FUNCTION "CENTR. 4  POSTERIORE SX" : VOID
TITLE =
VERSION : 0.1

BEGIN
NETWORK
TITLE =LETTURA STATUS WORD DA DRIVE
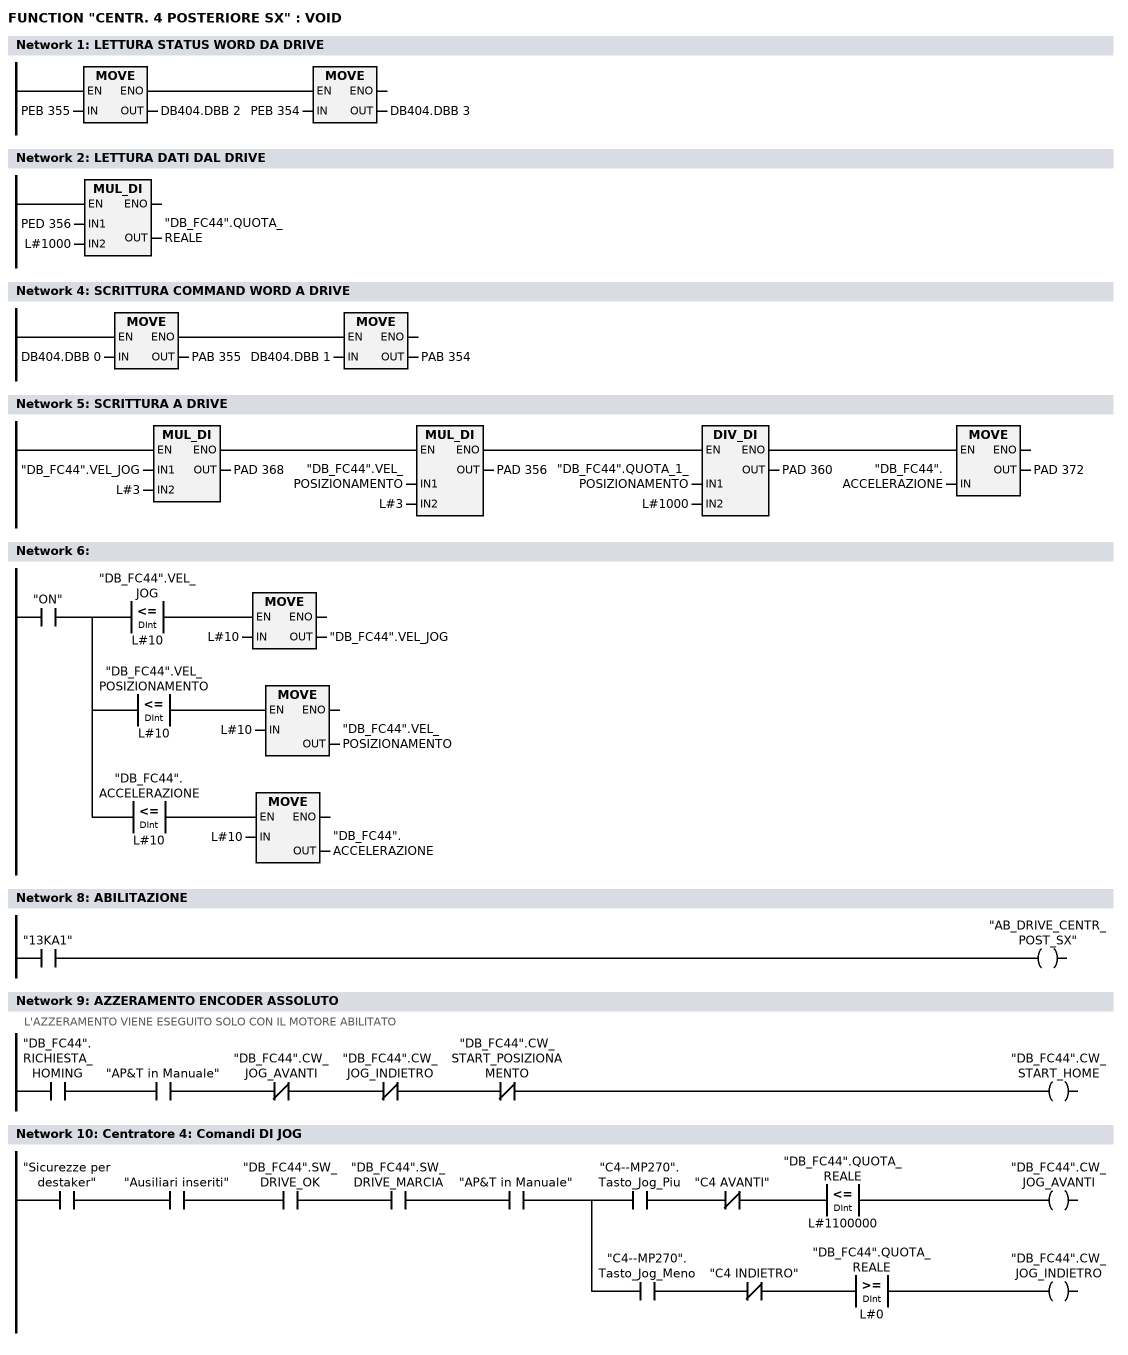
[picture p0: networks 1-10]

      U(    ;
      L     PEB  355;
      T     DB404.DBB    2;
      SET   ;
      SAVE  ;
      CLR   ;
      U     BIE;
      )     ;
      SPBNB _001;
      L     PEB  354;
      T     DB404.DBB    3;
_001: NOP   0;
NETWORK
TITLE =LETTURA DATI DAL DRIVE

      L     PED  356;
      L     L#1000;
      *D    ;
      T     "DB_FC44".QUOTA_REALE;
      NOP   0;
NETWORK
TITLE =

NETWORK
TITLE =SCRITTURA COMMAND WORD A DRIVE

      U(    ;
      L     DB404.DBB    0;
      T     PAB  355;
      SET   ;
      SAVE  ;
      CLR   ;
      U     BIE;
      )     ;
      SPBNB _002;
      L     DB404.DBB    1;
      T     PAB  354;
_002: NOP   0;
NETWORK
TITLE =SCRITTURA A DRIVE

      U(    ;
      U(    ;
      U(    ;
      L     "DB_FC44".VEL_JOG;
      L     L#3;
      *D    ;
      T     PAD  368;
      UN    OV;
      SAVE  ;
      CLR   ;
      U     BIE;
      )     ;
      SPBNB _003;
      L     "DB_FC44".VEL_POSIZIONAMENTO;
      L     L#3;
      *D    ;
      T     PAD  356;
      UN    OV;
      SAVE  ;
      CLR   ;
_003: U     BIE;
      )     ;
      SPBNB _004;
      L     "DB_FC44".QUOTA_1_POSIZIONAMENTO;
      L     L#1000;
      /D    ;
      T     PAD  360;
      UN    OV;
      SAVE  ;
      CLR   ;
_004: U     BIE;
      )     ;
      SPBNB _005;
      L     "DB_FC44".ACCELERAZIONE;
      T     PAD  372;
_005: NOP   0;
NETWORK
TITLE =

      U     "ON";
      =     L      0.0;
      U     L      0.0;
      U(    ;
      L     "DB_FC44".VEL_JOG;
      L     L#10;
      <=D   ;
      )     ;
      SPBNB _006;
      L     L#10;
      T     "DB_FC44".VEL_JOG;
_006: NOP   0;
      U     L      0.0;
      U(    ;
      L     "DB_FC44".VEL_POSIZIONAMENTO;
      L     L#10;
      <=D   ;
      )     ;
      SPBNB _007;
      L     L#10;
      T     "DB_FC44".VEL_POSIZIONAMENTO;
_007: NOP   0;
      U     L      0.0;
      U(    ;
      L     "DB_FC44".ACCELERAZIONE;
      L     L#10;
      <=D   ;
      )     ;
      SPBNB _008;
      L     L#10;
      T     "DB_FC44".ACCELERAZIONE;
_008: NOP   0;
NETWORK
TITLE =

NETWORK
TITLE =ABILITAZIONE

      U     "13KA1";
      =     "AB_DRIVE_CENTR_POST_SX";
NETWORK
TITLE =AZZERAMENTO ENCODER ASSOLUTO
//L'AZZERAMENTO VIENE ESEGUITO SOLO CON IL MOTORE ABILITATO
      U     "DB_FC44".RICHIESTA_HOMING;
      U     "AP&T in Manuale";
      UN    "DB_FC44".CW_JOG_AVANTI;
      UN    "DB_FC44".CW_JOG_INDIETRO;
      UN    "DB_FC44".CW_START_POSIZIONAMENTO;
      =     "DB_FC44".CW_START_HOME;
NETWORK
TITLE =Centratore 4: Comandi DI JOG

      U     "Sicurezze per destaker";
      U     "Ausiliari inseriti";
      U     "DB_FC44".SW_DRIVE_OK;
      U     "DB_FC44".SW_DRIVE_MARCIA;
      U     "AP&T in Manuale";
      =     L      0.0;
      U     L      0.0;
      U     "C4--MP270".Tasto_Jog_Piu;
      UN    "C4 AVANTI";
      U(    ;
      L     "DB_FC44".QUOTA_REALE;
      L     L#1100000;
      <=D   ;
      )     ;
      =     "DB_FC44".CW_JOG_AVANTI;
      U     L      0.0;
      U     "C4--MP270".Tasto_Jog_Meno;
      UN    "C4 INDIETRO";
      U(    ;
      L     "DB_FC44".QUOTA_REALE;
      L     L#0;
      >=D   ;
      )     ;
      =     "DB_FC44".CW_JOG_INDIETRO;
NETWORK
TITLE =Centratore 4: Posizioni

      U     "ON";
      =     L      0.0;
      U     L      0.0;
      U(    ;
      L     "DB_FC44".QUOTA_REALE;
      L     L#100;
      <=D   ;
      )     ;
      U(    ;
      L     "DB_FC44".QUOTA_REALE;
      L     L#-100;
      >=D   ;
      )     ;
      =     "C4: Asse in pos.0";
      U(    ;
      U(    ;
      U     L      0.0;
      SPBNB _009;
      L     "MATRICOLA ATTUALE".C4_Posizione_1;
      L     L#100;
      -D    ;
      T     "CONFRONTI CENTRATORI".C4_Pos_1_Min;
      UN    OV;
      SAVE  ;
      CLR   ;
_009: U     BIE;
      )     ;
      SPBNB _00a;
      L     "MATRICOLA ATTUALE".C4_Posizione_1;
      L     L#200;
      +D    ;
      T     "CONFRONTI CENTRATORI".C4_Pos_1_Max;
      UN    OV;
      SAVE  ;
      CLR   ;
_00a: U     BIE;
      )     ;
      U(    ;
      L     "DB_FC44".QUOTA_REALE;
      L     "CONFRONTI CENTRATORI".C4_Pos_1_Min;
      >=D   ;
      )     ;
      U(    ;
      L     "DB_FC44".QUOTA_REALE;
      L     "CONFRONTI CENTRATORI".C4_Pos_1_Max;
      <=D   ;
      )     ;
      =     "C4: Asse in pos.1";
      U(    ;
      U(    ;
      U     L      0.0;
      SPBNB _00b;
      L     "MATRICOLA ATTUALE".C4_Posizione_2;
      L     L#100;
      -D    ;
      T     "CONFRONTI CENTRATORI".C4_Pos_2_Min;
      UN    OV;
      SAVE  ;
      CLR   ;
_00b: U     BIE;
      )     ;
      SPBNB _00c;
      L     "MATRICOLA ATTUALE".C4_Posizione_2;
      L     L#50000;
      +D    ;
      T     "CONFRONTI CENTRATORI".C4_Pos_2_Max;
      UN    OV;
      SAVE  ;
      CLR   ;
_00c: U     BIE;
      )     ;
      U(    ;
      L     "DB_FC44".QUOTA_REALE;
      L     "CONFRONTI CENTRATORI".C4_Pos_2_Min;
      >=D   ;
      )     ;
      UN    "C4: Asse in pos.3";
      UN    "C4: Asse in pos.4";
      =     "C4: Asse in pos.2";
      U(    ;
      U(    ;
      U     L      0.0;
      SPBNB _00d;
      L     "MATRICOLA ATTUALE".C4_Posizione_3;
      L     L#100;
      -D    ;
      T     "CONFRONTI CENTRATORI".C4_Pos_3_Min;
      UN    OV;
      SAVE  ;
      CLR   ;
_00d: U     BIE;
      )     ;
      SPBNB _00e;
      L     "MATRICOLA ATTUALE".C4_Posizione_3;
      L     L#50000;
      +D    ;
      T     "CONFRONTI CENTRATORI".C4_Pos_3_Max;
      UN    OV;
      SAVE  ;
      CLR   ;
_00e: U     BIE;
      )     ;
      U(    ;
      L     "DB_FC44".QUOTA_REALE;
      L     "CONFRONTI CENTRATORI".C4_Pos_3_Min;
      >=D   ;
      )     ;
      UN    "C4: Asse in pos.4";
      =     "C4: Asse in pos.3";
      U(    ;
      U(    ;
      U     L      0.0;
      SPBNB _00f;
      L     "MATRICOLA ATTUALE".C4_Posizione_4;
      L     L#100;
      -D    ;
      T     "CONFRONTI CENTRATORI".C4_Pos_4_Min;
      UN    OV;
      SAVE  ;
      CLR   ;
_00f: U     BIE;
      )     ;
      SPBNB _010;
      L     "MATRICOLA ATTUALE".C4_Posizione_4;
      L     L#100;
      +D    ;
      T     "CONFRONTI CENTRATORI".C4_Pos_4_Max;
      UN    OV;
      SAVE  ;
      CLR   ;
_010: U     BIE;
      )     ;
      U(    ;
      L     "DB_FC44".QUOTA_REALE;
      L     "CONFRONTI CENTRATORI".C4_Pos_4_Min;
      >=D   ;
      )     ;
      U(    ;
      L     "DB_FC44".QUOTA_REALE;
      L     "CONFRONTI CENTRATORI".C4_Pos_4_Max;
      <=D   ;
      )     ;
      =     "C4: Asse in pos.4";
NETWORK
TITLE =Centratore 4: consenso abilitazione passi
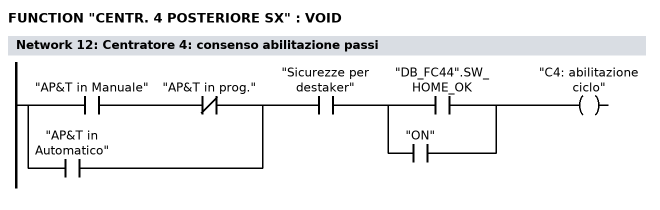
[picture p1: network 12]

      U(    ;
      U     "AP&T in Manuale";
      UN    "AP&T in prog.";
      O     "AP&T in Automatico";
      )     ;
      U     "Sicurezze per destaker";
      U(    ;
      O     "DB_FC44".SW_HOME_OK;
      O     "ON";
      )     ;
      =     "C4: abilitazione ciclo";
NETWORK
TITLE =Centratore 4: comando avvicinamento  (centraggi aperti)

      U(    ;
      U(    ;
      O     "Comando apre centraggi";
      O     "C4--MP270".Tasto_Indietro;
      O     ;
      U     "Apertura centratori";
      U(    ;
      O     "Centratori a riposo";
      O     "Centratori tutti chiusi";
      )     ;
      )     ;
      UN    "C4: Asse in pos.1";
      UN    "C4: comando arrivo";
      UN    "C4: comando a riposo";
      U     "C4: abilitazione ciclo";
      L     S5T#100MS;
      SE    T    190;
      NOP   0;
      NOP   0;
      NOP   0;
      U     T    190;
      )     ;
      S     "C4: comando avvicinam";
      U(    ;
      O     "C4: Asse in pos.1";
      O(    ;
      U(    ;
      O     "Ripristino centratori";
      O     "Comando riposo centraggi";
      O     "C4--MP270".Tasto_Riposo;
      )     ;
      FP    "C4: one shot 1";
      )     ;
      )     ;
      R     "C4: comando avvicinam";
      NOP   0;
NETWORK
TITLE =Centratore 4: comando arrivo (centraggi chiusi)

      U(    ;
      U(    ;
      O     "Comando chiude centraggi";
      O     "C4--MP270".Tasto_Avanti;
      O     ;
      U     "Chiusura centratori";
      U(    ;
      O     "Centratori tutti aperti";
      O     "Centratori a riposo";
      )     ;
      )     ;
      UN    "C4: Asse in pos.4";
      UN    "C4: comando avvicinam";
      UN    "C4: comando a riposo";
      U     "C4: abilitazione ciclo";
      L     S5T#100MS;
      SE    T    191;
      NOP   0;
      NOP   0;
      NOP   0;
      U     T    191;
      )     ;
      S     "C4: comando arrivo";
      U(    ;
      O     "C4: Asse in pos.4";
      O(    ;
      U(    ;
      O     "Ripristino centratori";
      O     "Comando riposo centraggi";
      O     "C4--MP270".Tasto_Riposo;
      )     ;
      FP    "C4: one shot 2";
      )     ;
      )     ;
      R     "C4: comando arrivo";
      NOP   0;
NETWORK
TITLE =Centratore 4: comando automatico centraggi a riposo

      U(    ;
      U(    ;
      O     "Comando riposo centraggi";
      O     "C4--MP270".Tasto_Riposo;
      )     ;
      UN    "C4: Asse in pos.0";
      UN    "C4: comando avvicinam";
      UN    "C4: comando arrivo";
      U     "C4: abilitazione ciclo";
      L     S5T#100MS;
      SE    T    192;
      NOP   0;
      NOP   0;
      NOP   0;
      U     T    192;
      )     ;
      S     "C4: comando a riposo";
      U(    ;
      O     "C4: Asse in pos.0";
      O(    ;
      U     "Ripristino centratori";
      FP    "C4: one shot 3";
      )     ;
      )     ;
      R     "C4: comando a riposo";
      NOP   0;
NETWORK
TITLE =Centratore 4: quote impostate per posizioni

      U     "ON";
      =     L      0.0;
      U(    ;
      U(    ;
      U     L      0.0;
      U     "C4: comando a riposo";
      UN    "C4: Asse in pos.0";
      SPBNB _011;
      L     0;
      T     "DB_FC44".QUOTA_1_POSIZIONAMENTO;
      SET   ;
      SAVE  ;
      CLR   ;
_011: U     BIE;
      )     ;
      SPBNB _012;
      L     L#150;
      T     "DB_FC44".VEL_POSIZIONAMENTO;
      SET   ;
      SAVE  ;
      CLR   ;
_012: U     BIE;
      )     ;
      SPBNB _013;
      L     L#1000;
      T     "DB_FC44".ACCELERAZIONE;
      SET   ;
      SAVE  ;
      CLR   ;
_013: U     BIE;
      =     "C4: Quote pronte pos.0";
      U(    ;
      U(    ;
      U     L      0.0;
      U     "C4: comando avvicinam";
      UN    "C4: Asse in pos.1";
      SPBNB _014;
      L     "MATRICOLA ATTUALE".C4_Posizione_1;
      T     "DB_FC44".QUOTA_1_POSIZIONAMENTO;
      SET   ;
      SAVE  ;
      CLR   ;
_014: U     BIE;
      )     ;
      SPBNB _015;
      L     "MATRICOLA ATTUALE".C4_Velocita_1;
      T     "DB_FC44".VEL_POSIZIONAMENTO;
      SET   ;
      SAVE  ;
      CLR   ;
_015: U     BIE;
      )     ;
      SPBNB _016;
      L     "MATRICOLA ATTUALE".C4_Accell_1;
      T     "DB_FC44".ACCELERAZIONE;
      SET   ;
      SAVE  ;
      CLR   ;
_016: U     BIE;
      =     "C4: Quote pronte pos.1";
      U     L      0.0;
      U     "C4: comando arrivo";
      =     L      0.1;
      U(    ;
      U(    ;
      U     L      0.1;
      UN    "C4: Asse in pos.2";
      SPBNB _017;
      L     "MATRICOLA ATTUALE".C4_Posizione_4;
      T     "DB_FC44".QUOTA_1_POSIZIONAMENTO;
      SET   ;
      SAVE  ;
      CLR   ;
_017: U     BIE;
      )     ;
      SPBNB _018;
      L     "MATRICOLA ATTUALE".C4_Velocita_2;
      T     "DB_FC44".VEL_POSIZIONAMENTO;
      SET   ;
      SAVE  ;
      CLR   ;
_018: U     BIE;
      )     ;
      SPBNB _019;
      L     "MATRICOLA ATTUALE".C4_Accell_2;
      T     "DB_FC44".ACCELERAZIONE;
      SET   ;
      SAVE  ;
      CLR   ;
_019: U     BIE;
      S     "C4: Quote pronte pos.2";
      U     L      0.1;
      U     "C4: Quote pronte pos.2";
      UN    "C4: Reset start pos.2";
      L     S5T#1S;
      SE    "C4: ritardo P2";
      NOP   0;
      NOP   0;
      NOP   0;
      U     "C4: ritardo P2";
      S     "C4: Reset start pos.2";
      R     "C4: Quote pronte pos.2";
      U     L      0.0;
      U     "C4: comando arrivo";
      =     L      0.1;
      U(    ;
      U(    ;
      U(    ;
      U     L      0.1;
      U     "C4: Asse in pos.2";
      UN    "C4: Asse in pos.3";
      SPBNB _01a;
      L     "MATRICOLA ATTUALE".C4_Posizione_4;
      T     "DB_FC44".QUOTA_1_POSIZIONAMENTO;
      SET   ;
      SAVE  ;
      CLR   ;
_01a: U     BIE;
      )     ;
      SPBNB _01b;
      L     "MATRICOLA ATTUALE".C4_Velocita_3;
      T     "DB_FC44".VEL_POSIZIONAMENTO;
      SET   ;
      SAVE  ;
      CLR   ;
_01b: U     BIE;
      )     ;
      SPBNB _01c;
      L     "MATRICOLA ATTUALE".C4_Accell_3;
      T     "DB_FC44".ACCELERAZIONE;
      SET   ;
      SAVE  ;
      CLR   ;
_01c: U     BIE;
      )     ;
      U     "C4: Reset start pos.2";
      S     "C4: Quote pronte pos.3";
      R     "C4: Reset start pos.2";
      U     L      0.1;
      U     "C4: Quote pronte pos.3";
      L     S5T#500MS;
      SE    "C4: ritardo P3";
      NOP   0;
      NOP   0;
      NOP   0;
      U     "C4: ritardo P3";
      S     "C4: Reset start pos.3";
      R     "C4: Quote pronte pos.3";
      U     L      0.0;
      U     "C4: comando arrivo";
      =     L      0.1;
      U(    ;
      U(    ;
      U(    ;
      U     L      0.1;
      U     "C4: Asse in pos.3";
      UN    "C4: Asse in pos.4";
      SPBNB _01d;
      L     "MATRICOLA ATTUALE".C4_Posizione_4;
      T     "DB_FC44".QUOTA_1_POSIZIONAMENTO;
      SET   ;
      SAVE  ;
      CLR   ;
_01d: U     BIE;
      )     ;
      SPBNB _01e;
      L     "MATRICOLA ATTUALE".C4_Velocita_4;
      T     "DB_FC44".VEL_POSIZIONAMENTO;
      SET   ;
      SAVE  ;
      CLR   ;
_01e: U     BIE;
      )     ;
      SPBNB _01f;
      L     "MATRICOLA ATTUALE".C4_Accell_4;
      T     "DB_FC44".ACCELERAZIONE;
      SET   ;
      SAVE  ;
      CLR   ;
_01f: U     BIE;
      )     ;
      U     "C4: Reset start pos.3";
      S     "C4: Quote pronte pos.4";
      R     "C4: Reset start pos.3";
      U     L      0.1;
      U     "C4: Quote pronte pos.4";
      L     S5T#500MS;
      SE    "C4: ritardo P4";
      NOP   0;
      NOP   0;
      NOP   0;
      U     "C4: ritardo P4";
      S     "C4: Reset start pos.4";
      R     "C4: Quote pronte pos.4";
NETWORK
TITLE =Centratore 4: reset impostate
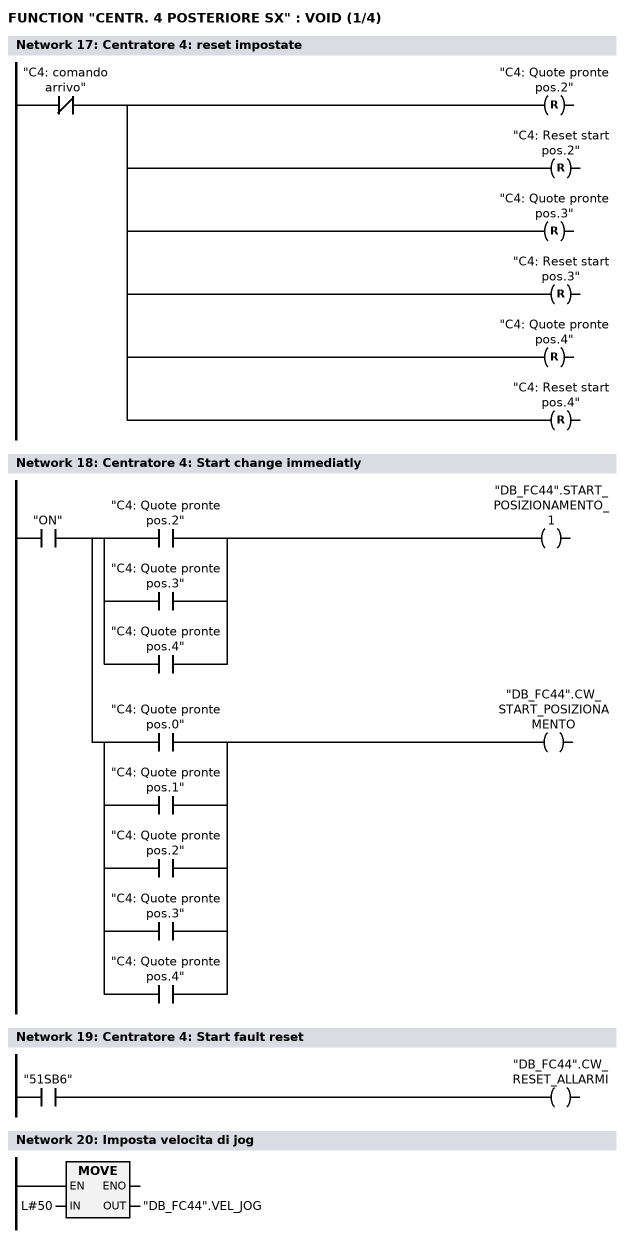
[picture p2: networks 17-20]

      UN    "C4: comando arrivo";
      R     "C4: Quote pronte pos.2";
      R     "C4: Reset start pos.2";
      R     "C4: Quote pronte pos.3";
      R     "C4: Reset start pos.3";
      R     "C4: Quote pronte pos.4";
      R     "C4: Reset start pos.4";
NETWORK
TITLE =Centratore 4: Start change immediatly

      U     "ON";
      =     L      0.0;
      U     L      0.0;
      U(    ;
      O     "C4: Quote pronte pos.2";
      O     "C4: Quote pronte pos.3";
      O     "C4: Quote pronte pos.4";
      )     ;
      =     "DB_FC44".START_POSIZIONAMENTO_1;
      U     L      0.0;
      U(    ;
      O     "C4: Quote pronte pos.0";
      O     "C4: Quote pronte pos.1";
      O     "C4: Quote pronte pos.2";
      O     "C4: Quote pronte pos.3";
      O     "C4: Quote pronte pos.4";
      )     ;
      =     "DB_FC44".CW_START_POSIZIONAMENTO;
NETWORK
TITLE =Centratore 4: Start fault reset

      U     "51SB6";
      =     "DB_FC44".CW_RESET_ALLARMI;
NETWORK
TITLE =Imposta velocita di jog

      L     L#50;
      T     "DB_FC44".VEL_JOG;
      NOP   0;
NETWORK
TITLE =Centratore 4: Drive Enable ok
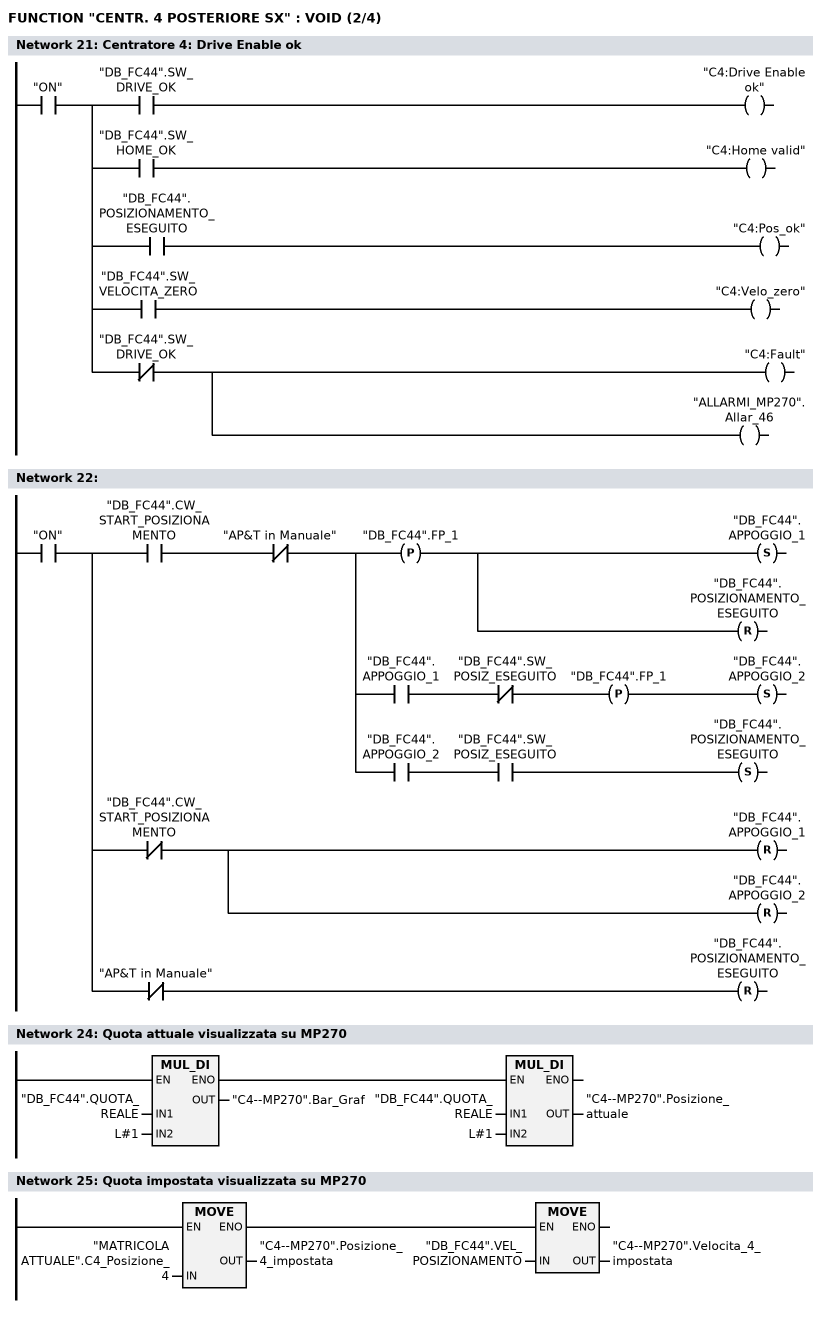
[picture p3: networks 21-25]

      U     "ON";
      =     L      0.0;
      U     L      0.0;
      U     "DB_FC44".SW_DRIVE_OK;
      =     "C4:Drive Enable ok";
      U     L      0.0;
      U     "DB_FC44".SW_HOME_OK;
      =     "C4:Home valid";
      U     L      0.0;
      U     "DB_FC44".POSIZIONAMENTO_ESEGUITO;
      =     "C4:Pos_ok";
      U     L      0.0;
      U     "DB_FC44".SW_VELOCITA_ZERO;
      =     "C4:Velo_zero";
      U     L      0.0;
      UN    "DB_FC44".SW_DRIVE_OK;
      =     "C4:Fault";
      =     "ALLARMI_MP270".Allar_46;
NETWORK
TITLE =

      U     "ON";
      =     L      0.0;
      U     L      0.0;
      U     "DB_FC44".CW_START_POSIZIONAMENTO;
      UN    "AP&T in Manuale";
      =     L      0.1;
      U     L      0.1;
      FP    "DB_FC44".FP_1;
      S     "DB_FC44".APPOGGIO_1;
      R     "DB_FC44".POSIZIONAMENTO_ESEGUITO;
      U     L      0.1;
      U     "DB_FC44".APPOGGIO_1;
      UN    "DB_FC44".SW_POSIZ_ESEGUITO;
      FP    "DB_FC44".FP_1;
      S     "DB_FC44".APPOGGIO_2;
      U     L      0.1;
      U     "DB_FC44".APPOGGIO_2;
      U     "DB_FC44".SW_POSIZ_ESEGUITO;
      S     "DB_FC44".POSIZIONAMENTO_ESEGUITO;
      U     L      0.0;
      UN    "DB_FC44".CW_START_POSIZIONAMENTO;
      R     "DB_FC44".APPOGGIO_1;
      R     "DB_FC44".APPOGGIO_2;
      U     L      0.0;
      UN    "AP&T in Manuale";
      R     "DB_FC44".POSIZIONAMENTO_ESEGUITO;
NETWORK
TITLE =

NETWORK
TITLE =Quota attuale visualizzata su MP270

      U(    ;
      L     "DB_FC44".QUOTA_REALE;
      L     L#1;
      *D    ;
      T     "C4--MP270".Bar_Graf;
      UN    OV;
      SAVE  ;
      CLR   ;
      U     BIE;
      )     ;
      SPBNB _020;
      L     "DB_FC44".QUOTA_REALE;
      L     L#1;
      *D    ;
      T     "C4--MP270".Posizione_attuale;
_020: NOP   0;
NETWORK
TITLE =Quota impostata visualizzata su MP270

      U(    ;
      L     "MATRICOLA ATTUALE".C4_Posizione_4;
      T     "C4--MP270".Posizione_4_impostata;
      SET   ;
      SAVE  ;
      CLR   ;
      U     BIE;
      )     ;
      SPBNB _021;
      L     "DB_FC44".VEL_POSIZIONAMENTO;
      T     "C4--MP270".Velocita_4_impostata;
_021: NOP   0;
NETWORK
TITLE =Visualizza FC su MP270
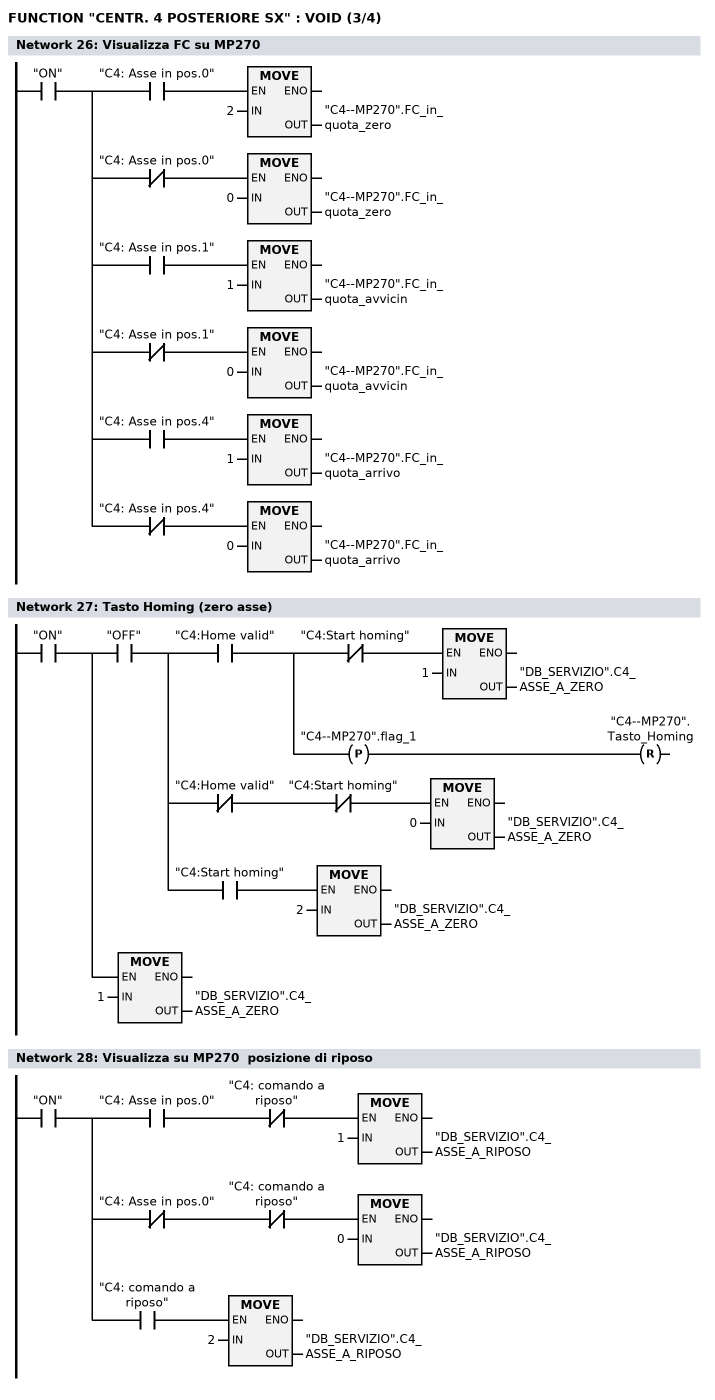
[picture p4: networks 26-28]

      U     "ON";
      =     L      0.0;
      U     L      0.0;
      U     "C4: Asse in pos.0";
      SPBNB _022;
      L     2;
      T     "C4--MP270".FC_in_quota_zero;
_022: NOP   0;
      U     L      0.0;
      UN    "C4: Asse in pos.0";
      SPBNB _023;
      L     0;
      T     "C4--MP270".FC_in_quota_zero;
_023: NOP   0;
      U     L      0.0;
      U     "C4: Asse in pos.1";
      SPBNB _024;
      L     1;
      T     "C4--MP270".FC_in_quota_avvicin;
_024: NOP   0;
      U     L      0.0;
      UN    "C4: Asse in pos.1";
      SPBNB _025;
      L     0;
      T     "C4--MP270".FC_in_quota_avvicin;
_025: NOP   0;
      U     L      0.0;
      U     "C4: Asse in pos.4";
      SPBNB _026;
      L     1;
      T     "C4--MP270".FC_in_quota_arrivo;
_026: NOP   0;
      U     L      0.0;
      UN    "C4: Asse in pos.4";
      SPBNB _027;
      L     0;
      T     "C4--MP270".FC_in_quota_arrivo;
_027: NOP   0;
NETWORK
TITLE =Tasto Homing (zero asse)

      U     "ON";
      =     L      0.0;
      U     L      0.0;
      U     "OFF";
      =     L      0.1;
      U     L      0.1;
      U     "C4:Home valid";
      =     L      0.2;
      U     L      0.2;
      UN    "C4:Start homing";
      SPBNB _028;
      L     1;
      T     "DB_SERVIZIO".C4_ASSE_A_ZERO;
_028: NOP   0;
      U     L      0.2;
      FP    "C4--MP270".flag_1;
      R     "C4--MP270".Tasto_Homing;
      U     L      0.1;
      UN    "C4:Home valid";
      UN    "C4:Start homing";
      SPBNB _029;
      L     0;
      T     "DB_SERVIZIO".C4_ASSE_A_ZERO;
_029: NOP   0;
      U     L      0.1;
      U     "C4:Start homing";
      SPBNB _02a;
      L     2;
      T     "DB_SERVIZIO".C4_ASSE_A_ZERO;
_02a: NOP   0;
      U     L      0.0;
      SPBNB _02b;
      L     1;
      T     "DB_SERVIZIO".C4_ASSE_A_ZERO;
_02b: NOP   0;
NETWORK
TITLE =Visualizza su MP270  posizione di riposo

      U     "ON";
      =     L      0.0;
      U     L      0.0;
      U     "C4: Asse in pos.0";
      UN    "C4: comando a riposo";
      SPBNB _02c;
      L     1;
      T     "DB_SERVIZIO".C4_ASSE_A_RIPOSO;
_02c: NOP   0;
      U     L      0.0;
      UN    "C4: Asse in pos.0";
      UN    "C4: comando a riposo";
      SPBNB _02d;
      L     0;
      T     "DB_SERVIZIO".C4_ASSE_A_RIPOSO;
_02d: NOP   0;
      U     L      0.0;
      U     "C4: comando a riposo";
      SPBNB _02e;
      L     2;
      T     "DB_SERVIZIO".C4_ASSE_A_RIPOSO;
_02e: NOP   0;
NETWORK
TITLE =Visualizza su MP270  posizione di avvicinamento
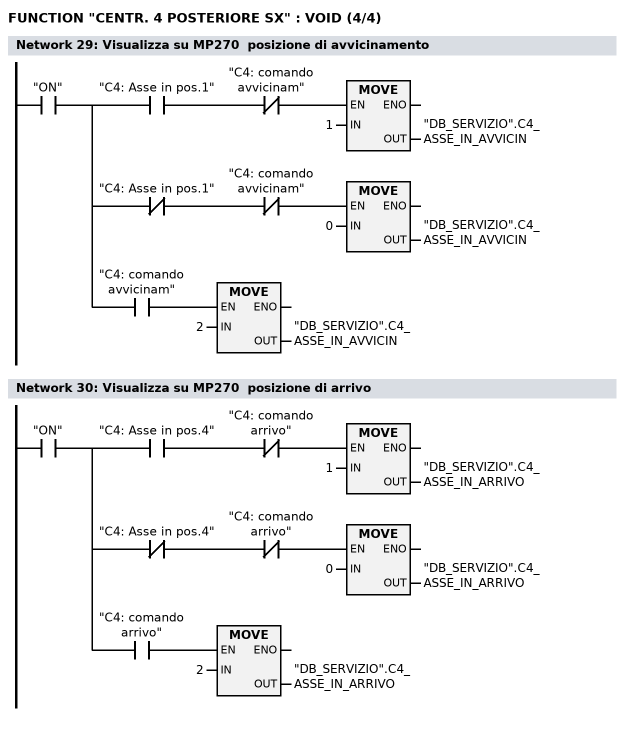
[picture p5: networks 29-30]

      U     "ON";
      =     L      0.0;
      U     L      0.0;
      U     "C4: Asse in pos.1";
      UN    "C4: comando avvicinam";
      SPBNB _02f;
      L     1;
      T     "DB_SERVIZIO".C4_ASSE_IN_AVVICIN;
_02f: NOP   0;
      U     L      0.0;
      UN    "C4: Asse in pos.1";
      UN    "C4: comando avvicinam";
      SPBNB _030;
      L     0;
      T     "DB_SERVIZIO".C4_ASSE_IN_AVVICIN;
_030: NOP   0;
      U     L      0.0;
      U     "C4: comando avvicinam";
      SPBNB _031;
      L     2;
      T     "DB_SERVIZIO".C4_ASSE_IN_AVVICIN;
_031: NOP   0;
NETWORK
TITLE =Visualizza su MP270  posizione di arrivo

      U     "ON";
      =     L      0.0;
      U     L      0.0;
      U     "C4: Asse in pos.4";
      UN    "C4: comando arrivo";
      SPBNB _032;
      L     1;
      T     "DB_SERVIZIO".C4_ASSE_IN_ARRIVO;
_032: NOP   0;
      U     L      0.0;
      UN    "C4: Asse in pos.4";
      UN    "C4: comando arrivo";
      SPBNB _033;
      L     0;
      T     "DB_SERVIZIO".C4_ASSE_IN_ARRIVO;
_033: NOP   0;
      U     L      0.0;
      U     "C4: comando arrivo";
      SPBNB _034;
      L     2;
      T     "DB_SERVIZIO".C4_ASSE_IN_ARRIVO;
_034: NOP   0;
END_FUNCTION

